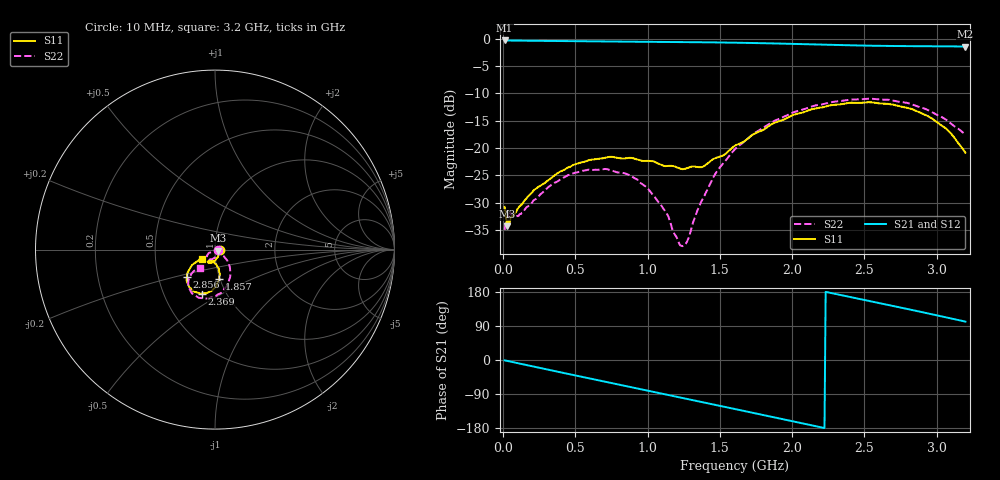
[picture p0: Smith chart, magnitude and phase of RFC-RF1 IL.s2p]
!Agilent Technologies,N5230A,MY45001650,A.07.50.48
!Agilent N5230A: A.07.50.48
!Date: Monday, December 05, 2022 16:01:44
!Correction: S11(Full 2 Port(1,2))
!S21(Full 2 Port(1,2))
!S12(Full 2 Port(1,2))
!S22(Full 2 Port(1,2))
!S2P File: Measurements: S11, S21, S12, S22:
# Hz S  dB  R 50
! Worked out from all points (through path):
!   400 points, 10 MHz to 3.2 GHz, reference 50 ohm
!   highest |S21| = -0.33 dB at 10 MHz (marker M1); lowest = -1.4 dB at 3.2 GHz (marker M2)
!   group delay of S21, straight-line fit = 224 ps
!   lowest |S11| = -34.4 dB at 25.99 MHz (marker M3), VSWR 1.04, Z = 51.8 - j0.657 ohm
!   |S11| at or under -10 dB: start of sweep to end of sweep
!   |S22| runs from -38.0 to -11.0 dB; largest |S21 - S12| = 0.001
!   S11 on the Smith chart (normalised r, x): 10 MHz: 1.06, -0.00; 1.857 GHz: 0.99, -0.33; 2.369 GHz: 0.77, -0.40; 2.856 GHz: 0.70, -0.23; 3.2 GHz: 0.86, -0.09
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1e7  -30.77 -3.6  -0.33 -0.9  -0.33 -0.9  -34.97 -1.3
2.598997e7  -34.35 -19.3  -0.35 -2.1  -0.35 -2.1  -31.42 -11.2
3.398496e7  -33.24 -18.2  -0.34 -2.8  -0.34 -2.8  -32.69 -14.4
4.197995e7  -34.17 -19.6  -0.35 -3.5  -0.35 -3.5  -32.67 -15.2
4.997494e7  -32.91 -20.5  -0.34 -4.2  -0.34 -4.1  -31.78 -16.2
1.059398e8  -30.91 -39.7  -0.37 -8.8  -0.37 -8.8  -32.42 -42.5
2.178697e8  -27.59 -65.3  -0.39 -18.0  -0.39 -18.0  -29.46 -76.9
3.537845e8  -25.04 -85.7  -0.42 -29.0  -0.42 -29.0  -26.37 -96.2
5.456642e8  -22.61 -103.5  -0.47 -44.4  -0.47 -44.4  -24.16 -117.4
8.654637e8  -21.82 -119.4  -0.55 -70.0  -0.55 -70.0  -24.85 -142.4
1.081328e9  -22.94 -118.1  -0.59 -87.2  -0.59 -87.2  -30.01 -148.9
1.225238e9  -23.78 -110.1  -0.62 -98.7  -0.62 -98.7  -37.81 -108.5
1.257218e9  -23.81 -108.1  -0.63 -101.3  -0.63 -101.3  -37.72 -83.9
1.449098e9  -22.10 -89.3  -0.68 -116.8  -0.68 -116.8  -25.66 -35.3
1.608997e9  -19.52 -79.0  -0.74 -129.7  -0.74 -129.7  -20.11 -43.5
1.856842e9  -15.69 -81.8  -0.87 -149.9  -0.87 -149.9  -15.35 -60.1
2.136667e9  -12.92 -93.3  -1.05 -172.5  -1.04 -172.5  -12.40 -80.6
2.368521e9  -11.86 -106.4  -1.19 168.9  -1.19 169.0  -11.27 -97.3
2.672331e9  -11.96 -125.1  -1.34 144.7  -1.33 144.7  -11.19 -117.5
2.856216e9  -13.18 -135.5  -1.37 129.9  -1.36 129.9  -12.27 -128.0
3.07208e9  -16.58 -146.3  -1.41 112.1  -1.40 112.1  -14.93 -134.6
3.2e9  -20.86 -146.1  -1.44 101.3  -1.44 101.3  -17.56 -130.7
